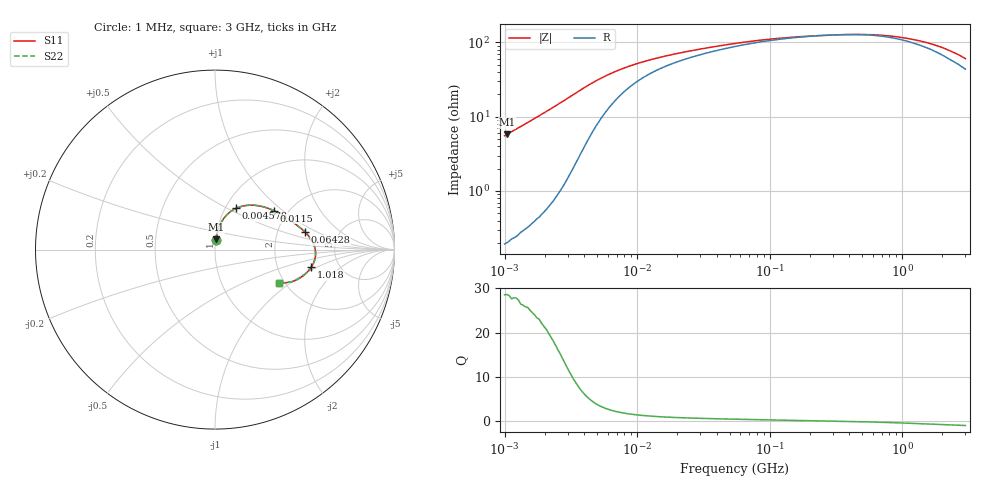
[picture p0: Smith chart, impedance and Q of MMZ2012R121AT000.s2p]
! S-parameter Generated by TDK Corporation
! Copyright(C) 2016 TDK Corporation.
! All Rights Reserved.
! TDK P/N: MMZ2012R121AT000 (Chip Beads)
! Property: |Z|=120¶ at 100MHz
! Size(LxWxT): 2x1.25x0.85mm, 0.079x0.049x0.033inches
! Model Type: s2p (Touchstone File Format Version 1.0)
! Frequency: DC=Yes Start=1MHz Stop=3000MHz 202points Log-sweep
! Note: This model was converted from impedance.
! Model Generated on May. 16, 2016
! Hash(MD5):
! Port Assignments:
!  1 ---@@@--- 2
! Applicable Conditions:
!  Temperature = 25 degC
!  DC Bias Current = 0 A
!  Small Signal Operation
! Terms and conditions regarding TDK Simulation Models
! (1)This simulation model is being provided solely for informational purposes. Please refer to the specifications of the products in terms of detailed characteristics of such products.
! (2)In no event shall TDK Corporation of any of its subsidiaries be liable for any loss or damage arising, directly or indirectly,
!  From any information contained in this simulation model, including, but not limited to loss or damages arising from any inaccuracies, omissions or errors in connection with such information.
! (3)Any and all copyrights on this simulation model are owned by TDK Corporation.
!  Duplication or redistribution of this simulation model without prior written permission from TDK Corporation is prohibited.
! (4)This simulation model is subject to any modification or change without any prior notice.
! (5)Neither TDK Corporation nor any of its subsidiaries shall make any warranty, express or implied,
!  Including but not limited to the correctness, implied warranties of merchantability and fitness for a particular purpose with respect to this simulation models.
! (6)The use of this simulation model shall be deemed to have consented to the terms and conditions hereof.
# MHz S MA R 50
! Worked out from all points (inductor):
!   201 points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, 1 MHz to 3 GHz, reference 50 ohm
!   read as one part in series: L = 885 nH near 1.041 MHz
!   highest Q = 28.6 at 1.041 MHz (marker M1), where L = 882 nH
!   self-resonance near 341.3 MHz
!   S11 on the Smith chart (normalised r, x): 1 MHz: 1.00, +0.11; 4.578 MHz: 1.12, +0.55; 11.5 MHz: 1.70, +0.87; 64.28 MHz: 2.86, +0.76; 1.018 GHz: 3.14, -0.87; 3 GHz: 1.87, -0.83
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1  0.05526 84.8  0.9965 -3.2  0.9965 -3.2  0.05526 84.8
1.040844  0.05751 84.7  0.9963 -3.3  0.9963 -3.3  0.05751 84.7
1.682724  0.09356 82.3  0.9917 -5.4  0.9917 -5.4  0.09356 82.3
2.412589  0.1364 78.9  0.9828 -7.8  0.9828 -7.8  0.1364 78.9
3.067588  0.1765 74.8  0.9688 -10.1  0.9688 -10.1  0.1765 74.8
3.900413  0.2248 68.4  0.9408 -12.8  0.9408 -12.8  0.2248 68.4
4.57776  0.2585 62.9  0.9118 -14.6  0.9118 -14.6  0.2585 62.9
5.592179  0.2973 55.5  0.8671 -16.4  0.8671 -16.4  0.2973 55.5
6.83139  0.3305 48.3  0.8185 -17.6  0.8185 -17.6  0.3305 48.3
11.49534  0.3932 33.5  0.7061 -17.9  0.7061 -17.9  0.3932 33.5
14.61624  0.4147 28.5  0.6655 -17.3  0.6655 -17.3  0.4147 28.5
25.59965  0.4562 20.0  0.5923 -15.3  0.5923 -15.3  0.4562 20.0
54.77226  0.5024 12.4  0.5208 -12.0  0.5208 -12.0  0.5024 12.4
64.28402  0.5105 11.1  0.5088 -11.2  0.5088 -11.2  0.5105 11.1
213.6344  0.5506 3.0  0.4511 -3.7  0.4511 -3.7  0.5506 3.0
457.0858  0.5608 -2.1  0.4401 2.7  0.4401 2.7  0.5608 -2.1
800.5644  0.555 -7.5  0.4555 9.1  0.4555 9.1  0.555 -7.5
1017.911  0.5455 -10.3  0.4733 11.8  0.4733 11.8  0.5455 -10.3
1402.151  0.5247 -14.5  0.5093 15.0  0.5093 15.0  0.5247 -14.5
1855.641  0.4959 -18.9  0.5548 16.9  0.5548 16.9  0.4959 -18.9
2556.106  0.4412 -24.6  0.6263 17.0  0.6263 17.0  0.4412 -24.6
3000  0.4031 -27.6  0.6691 16.2  0.6691 16.2  0.4031 -27.6
